(* Logix 5000 AddOnInstructionDefinition export AKD_Response_Status_Words; software revision 20.04 *)

TYPE AKD_Status :   // All connections to the drive ethernet module are established and data is successfully transferring.
STRUCT
   Profile_In_Progress : BOOL;   // Profile Move In Progress
   Block_In_Execution : BOOL;   // Block In Execution
   On_Target_Position : BOOL;   // On Target Position (1=Current Position Equals Last Target Position)
   General_Fault : BOOL;   // General Fault
   Current_Direction : BOOL;   // Current Motor Direction (0=Reverse, 1=Forward)
   Home_Level : BOOL;   // Level of Home Input
   Reg_Level : BOOL;   // Level of Registration Input
   Enable : BOOL;   // State of Enable Output
   Fault_Input_Fault : BOOL;   // Fault Input Active
   Fwd_Limit : BOOL;   // Forward Input Active
   Rev_Limit : BOOL;   // Reverse Input Active
   Positive_Limit : BOOL;   // Positive Software Limit Exceeded
   Negative_Limit : BOOL;   // Negative Software Limit Exceeded
   FE_Fault : BOOL;   // Following Error Fault
   Block_Fault : BOOL;   // Block Execution Fault
   Load_Complete : BOOL;   // Command Message Successfully Loaded
END_STRUCT
END_TYPE

TYPE AKD_Control :   // Send Explicit Message
STRUCT
   Load_Data_Start_Profile : BOOL;   // Load Command Data / Start Profile Move
   Start_Block : BOOL;   // Execute Command block or block chain
   Incremental : BOOL;   // Incremental Position (0=Absolute, 1=Incremental)
   Direction : BOOL;   // Direction in Velocity Mode (0=Reverse, 1=Forward)
   Smooth_Stop : BOOL;   // Smooth / Controlled Stop w/ Deceleration
   Hard_Stop : BOOL;   // Hard / Immediate Stop
   Reg_Arm : BOOL;   // Arm the Registration Input
   Enable : BOOL;   // Enable Output
END_STRUCT
END_TYPE

TYPE AKD_Axis :   // Axis Data:
STRUCT
   Control : AKD_Control;   // Control bits to send to the drive
   Status : AKD_Status;   // Status bits received from the drive
   Input : AB:ETHERNET_MODULE_SINT_64Bytes:I:0;   // Data from the drive
   Output : AB:ETHERNET_MODULE_SINT_64Bytes:O:0;   // Data to the drive
   ResponseMsgType : SINT;   // Response type contained in latest IO response from drive. Used to check for errors
   CommandTimeout : INT;   // Time to allow for command response from drive. Dependent on scan rate and communicaiton rate
   PositionFeedback : DINT;   // Actual Position Value
   VelocityFeedback : DINT;   // Actual Velocity Value
END_STRUCT
END_TYPE

ADD_ON_INSTRUCTION AKD_Response_Status_Words   (* revision 2.0 *)
VAR_IN_OUT
   Axis : AKD_Axis; {required}
END_VAR
VAR_OUTPUT
   Profile_In_Progress_In_Motion : BOOL; {access Read Only, visible}
   Block_In_Execution : BOOL; {access Read Only, visible}
   In_Position : BOOL; {access Read Only, visible}
   General_Fault : BOOL; {access Read Only, visible}
   Current_Direction : BOOL; {access Read Only, visible}
   Homed : BOOL; {access Read Only, visible}
   Reserved_Bit_6_Status_Word1 : BOOL; {access Read Only, visible}
   Enabled : BOOL; {access Read Only, visible}
   Reserved_Bit_0_Status_Word2 : BOOL; {visible}
   Fwd_HW_Limit : BOOL; {access Read Only, visible}
   Neg_HW_Limit : BOOL; {access Read Only, visible}
   Positive_SW_Limit : BOOL; {access Read Only, visible}
   Negative_SW_Limit : BOOL; {access Read Only, visible}
   Reserved_Bit_5_Status_Word2 : BOOL; {visible}
   Reserved_Bit_6_Status_Word2 : BOOL; {visible}
   Load_Complete : BOOL; {access Read Only, visible}
   FE_Fault : BOOL; {access Read Only}
   Fault_Input_Fault : BOOL; {access Read Only}
   Block_Fault : BOOL; {access Read Only}
END_VAR

ROUTINE Logic   (* ladder *)
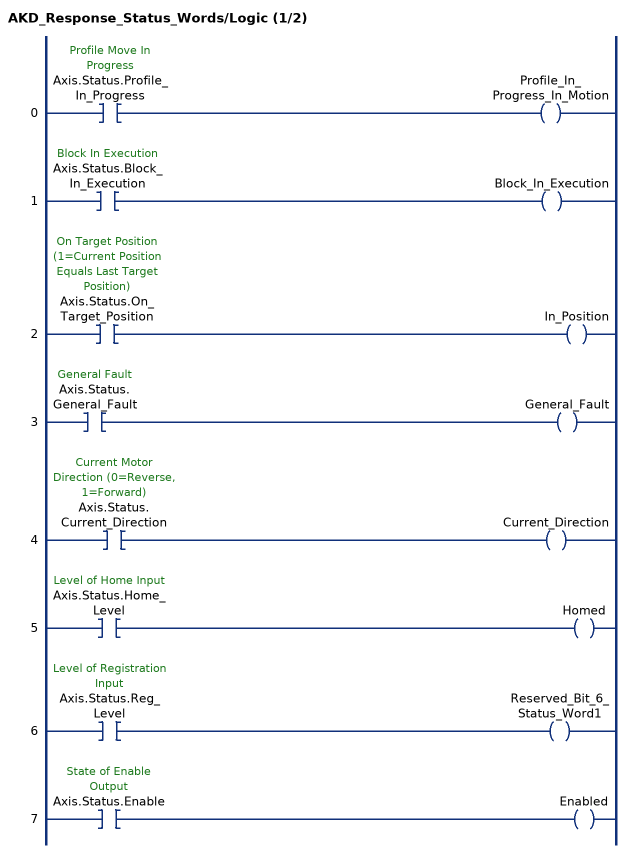
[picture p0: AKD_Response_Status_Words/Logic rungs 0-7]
   0: XIC(Axis.Status.Profile_In_Progress)OTE(Profile_In_Progress_In_Motion);
   1: XIC(Axis.Status.Block_In_Execution)OTE(Block_In_Execution);
   2: XIC(Axis.Status.On_Target_Position)OTE(In_Position);
   3: XIC(Axis.Status.General_Fault)OTE(General_Fault);
   4: XIC(Axis.Status.Current_Direction)OTE(Current_Direction);
   5: XIC(Axis.Status.Home_Level)OTE(Homed);
   6: XIC(Axis.Status.Reg_Level)OTE(Reserved_Bit_6_Status_Word1);
   7: XIC(Axis.Status.Enable)OTE(Enabled);
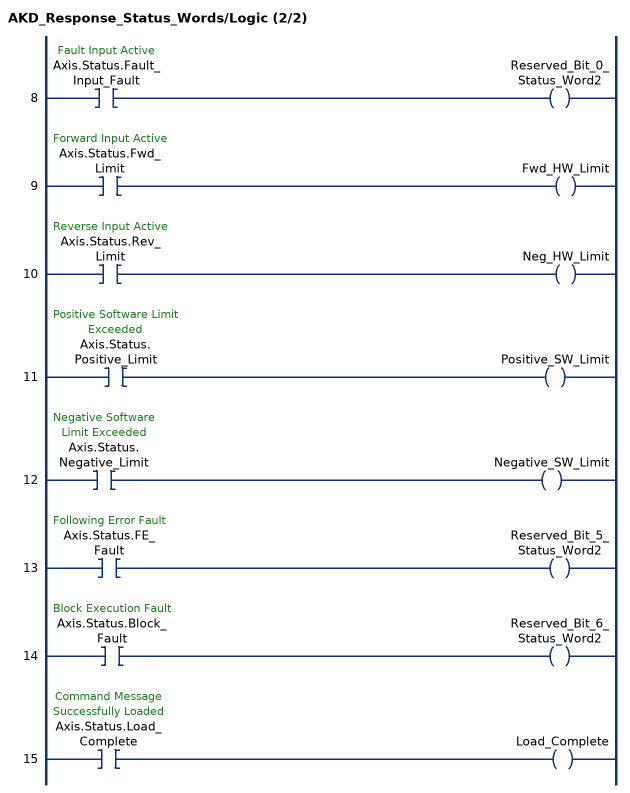
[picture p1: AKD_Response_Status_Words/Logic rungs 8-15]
   8: XIC(Axis.Status.Fault_Input_Fault)OTE(Reserved_Bit_0_Status_Word2);
   9: XIC(Axis.Status.Fwd_Limit)OTE(Fwd_HW_Limit);
   10: XIC(Axis.Status.Rev_Limit)OTE(Neg_HW_Limit);
   11: XIC(Axis.Status.Positive_Limit)OTE(Positive_SW_Limit);
   12: XIC(Axis.Status.Negative_Limit)OTE(Negative_SW_Limit);
   13: XIC(Axis.Status.FE_Fault)OTE(Reserved_Bit_5_Status_Word2);
   14: XIC(Axis.Status.Block_Fault)OTE(Reserved_Bit_6_Status_Word2);
   15: XIC(Axis.Status.Load_Complete)OTE(Load_Complete);
END_ROUTINE
END_ADD_ON_INSTRUCTION
